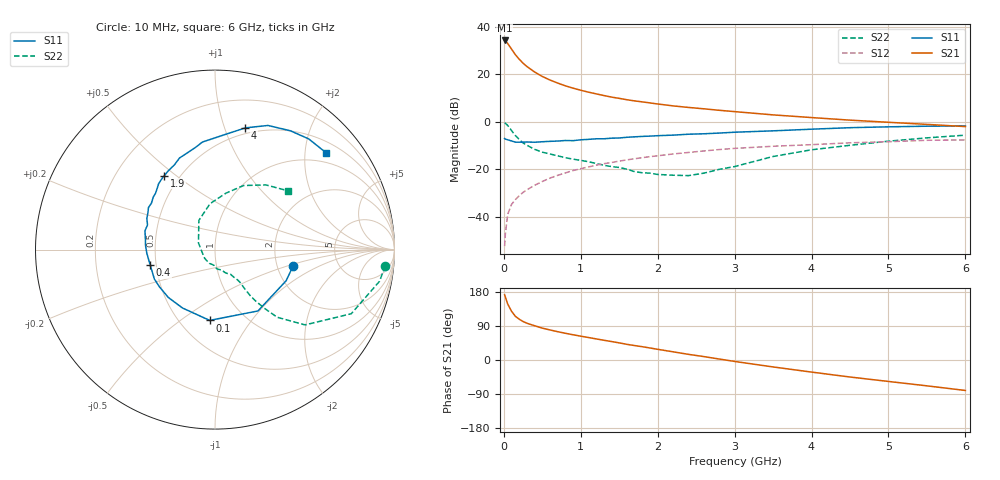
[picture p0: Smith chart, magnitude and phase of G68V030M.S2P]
! SIEMENS Small Signal Semiconductors
! BFG193
! Si NPN RF Bipolar Junction Transistor in SOT223
! VCE = 8 V  IC = 30 mA
! Common Emitter S-Parameters:  August  1996
# GHz  S  MA  R  50
!  f  S11  S21  S12  S22
! GHz  MAG  ANG  MAG  ANG  MAG  ANG  MAG  ANG
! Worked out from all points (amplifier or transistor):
!   36 points, 10 MHz to 6 GHz, reference 50 ohm
!   highest |S21| = 34.3 dB at 10 MHz (marker M1)
!   |S21| within 3 dB of that: start of sweep to 86.61 MHz
!   unconditionally stable (mu >= 1): 647 MHz to 2.489 GHz
!   at 250 MHz: K = 0.82, MSG = 27.2 dB, |S12| = -29.7 dB
!   at 1.4 GHz: K = 1.04, MAG = 12.5 dB, |S12| = -17.1 dB
!   at 6 GHz: K = 0.89, MSG = 2.8 dB, |S12| = -7.6 dB
!   S11 on the Smith chart (normalised r, x): 10 MHz: 2.45, -0.55; 100 MHz: 0.69, -0.65; 400 MHz: 0.46, -0.09; 1.9 GHz: 0.41, +0.45; 4 GHz: 0.44, +1.18; 6 GHz: 0.74, +2.47
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0.01  0.4447 -11.7  51.72 172.1  0.0024 88.0  0.9528 -5.5
0.02  0.4328 -23.6  50.53 166.2  0.0044 82.1  0.9335 -10.9
0.05  0.4173 -55.0  44.73 147.9  0.0112 71.7  0.8391 -25.2
0.1  0.3956 -94.3  34.03 128.6  0.0182 65.2  0.654 -39.9
0.15  0.3724 -119.1  25.91 115.3  0.023 61.8  0.5122 -47.4
0.2  0.3724 -134.3  20.84 107.6  0.0277 63.2  0.4252 -50.0
0.25  0.3726 -145.9  17.15 101.6  0.0326 63.1  0.3595 -51.8
0.3  0.3754 -154.1  14.61 97.0  0.037 64.2  0.3207 -52.6
0.4  0.3713 -166.8  11.2 90.4  0.046 64.8  0.2629 -52.8
0.5  0.3803 -176.9  9.02 84.1  0.0553 64.7  0.2292 -52.6
0.6  0.3876 176.7  7.588 79.3  0.0652 64.1  0.2096 -53.4
0.7  0.3934 170.5  6.548 74.7  0.0745 63.5  0.1921 -55.1
0.9  0.4005 159.9  5.114 66.6  0.094 60.3  0.1633 -57.7
1.1  0.4267 151.1  4.214 59.3  0.1118 57.3  0.1442 -65.1
1.4  0.4518 139.5  3.313 48.7  0.139 51.6  0.1141 -77.0
1.9  0.4996 124.5  2.499 31.7  0.1845 41.5  0.0829 -112.4
2.2  0.524 115.5  2.165 21.6  0.2101 34.6  0.075 -140.9
3.5  0.6451 84.7  1.399 -18.3  0.3054 4.2  0.186 118.9
4  0.699 76.0  1.229 -31.9  0.33 -5.5  0.2574 96.1
4.5  0.7519 66.9  1.084 -44.9  0.3611 -15.6  0.32 79.1
5.5  0.8079 49.8  0.882 -68.2  0.408 -38.8  0.4588 51.8
6  0.821 41.2  0.793 -80.4  0.4155 -52.3  0.523 38.7
